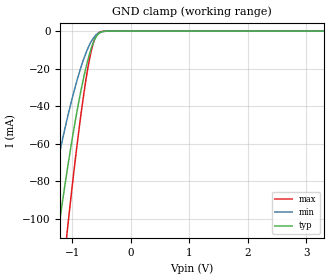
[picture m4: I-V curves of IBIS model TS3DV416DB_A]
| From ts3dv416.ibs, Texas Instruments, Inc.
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[Model]   TS3DV416DB_A
Model_type  Terminator
| variable   typ   min   max
C_comp   5.65pF   4.67pF   6.28pF
| C_tri-state   5.65pF   4.67pF   6.28pF
[Temperature Range]   40   100   -40
| Ambient temperature   25   85   -40
[Voltage range]   3.3   3   3.6
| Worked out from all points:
|   GND clamp passes 1 mA (typ) near -0.53 V on its own axis
[GND Clamp]
| TS3DV416DB_A
|   Voltage   I(typ)   I(min)   I(max)
-3.3V     -705.7mA   -513.3mA   -914.9mA
-1.48V    -164.7mA   -108.2mA   -233.4mA
-1.44V    -154.7mA   -101.3mA   -219.8mA
-1.23V    -105.2mA   -67.37mA   -151.1mA
-1.1V     -77.34mA   -48.81mA   -111.5mA
-1.07V    -71.28mA   -44.82mA   -102.7mA
-885mV    -37.45mA   -22.93mA   -52.99mA
-740mV    -16.44mA   -9.851mA   -21.3mA
-640mV    -6.256mA   -3.859mA   -6.596mA
-595mV    -3.318mA   -2.165mA   -2.921mA
-535mV    -1.105mA   -821.4uA   -692.5uA
3.3V      3.616nA    4.558nA    3.34nA
